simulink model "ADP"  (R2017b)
settings: Solver=FixedStepDiscrete  StartTime=0.0  StopTime=10.0  FixedStep=0.01  RelTol=1e-3  EnableMultiTasking=on
undefined symbols (not defined in the file): ADP050_RUNTIME_MS, ADP195_RUNTIME_MS, ADP_CONST100_NUMB, ADP_CONST2147483648_NUMB, ADP_CONST3_NUMB, ADP_CONST80_NUMB, ASWTYPE_FALSE, ASWTYPE_TRUE, CcADP_ABMDiagKL15DelayTi_ms, CcADP_ObcCmdto0Ti_ms, Enum_ADPStopChgReq, Enum_ISPDischgReq, Enum_LDPCC2St, Enum_MSMBMUState, Enum_ODPCCState, Enum_UDSPrjSel
libraries: AIWAYS_Powertrain_BMS_lib x68
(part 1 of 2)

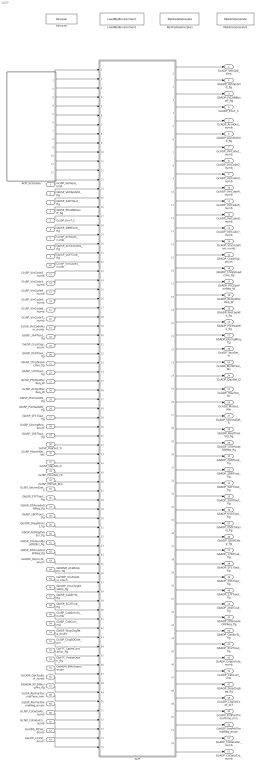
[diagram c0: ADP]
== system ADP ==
  GcISP_VehSpd_kmh : Inport
  GbISP_VehSpdVld_flg : Inport  Port=2
  GbISP_2ADTiout_flg : Inport  Port=3
  GbISP_PtCANBusoff_flg : Inport  Port=4
  GcISP_EnvT_C : Inport  Port=5
  GbISP_2BBTiout_flg : Inport  Port=6
  GcISP_AcmDist_numb : Inport  Port=7
  GbISP_AcmDistVld_flg : Inport  Port=8
  GbISP_2DFTiout_flg : Inport  Port=9
  GcISP_VinCode1_numb : Inport  Port=10
  GcISP_VinCode2_numb : Inport  Port=11
  GcISP_VinCode3_numb : Inport  Port=12
  GcISP_VinCode4_numb : Inport  Port=13
  GcISP_VinCode5_numb : Inport  Port=14
  GcISP_VinCode6_numb : Inport  Port=15
  GcISP_VinCode7_numb : Inport  Port=16
  GcISP_VinCodeNum_numb : Inport  Port=17
  GbISP_3AATiout_flg : Inport  Port=18
  GeISP_CrashSgl_enum : Inport  Port=19
  GbISP_050Tiout_flg : Inport  Port=20
  GbISP_ChrgStopActive_flg : Inport  Port=21
  GbISP_17DTiout_flg : Inport  Port=22
  GcISP_PTCOptPwrReq_W : Inport  Port=23
  GcISP_ACOptPwrReq_W : Inport  Port=24
  GbISP_PreCoolWk_flg : Inport  Port=25
  GbISP_PreHeatWk_flg : Inport  Port=26
  GbISP_2F1Tiout_flg : Inport  Port=27
  GeISP_DischgReq_enum : Inport  Port=28
  GbISP_195Tiout_flg : Inport  Port=29
  GcISP_YearSet_Yr : Inport  Port=30
  GcISP_MonthSet_Mn : Inport  Port=31
  GcISP_DaySet_D : Inport  Port=32
  GcISP_HourSet_Hr : Inport  Port=33
  GcISP_MinSet_Min : Inport  Port=34
  GcISP_SecondSet_S : Inport  Port=35
  GbISP_37FTiout_flg : Inport  Port=36
  GbISP_OTAmodeONReq_flg : Inport  Port=37
  GbISP_28DTiout_flg : Inport  Port=38
  GbVDP_DiagPermit_flg : Inport  Port=39
  GbISP_RcMsg050Err_flg : Inport  Port=40
  GbISP_ChkSumMsg050Err_flg : Inport  Port=41
  GbISP_OTAmodeOFFReq_flg : Inport  Port=42
  GeODP_ObcCcSt_enum : Inport  Port=43
  GbWSM_ACWkUpPrs_flg : Inport  Port=44
  GeVDP_VcuFalutLvl_enum : Inport  Port=45
  GbVDP_VcuChrgDisable_flg : Inport  Port=46
  GbISP_CabErrSt_flg : Inport  Port=47
  GbISP_3C2Tiout_flg : Inport  Port=48
  GcISP_CabErrInfo_numb : Inport  Port=49
  GcISP_CabCurr_mA : Inport  Port=50
  GeISP_StopChgReq_enum : Inport  Port=51
  GcISP_ChgSOCset_pct : Inport  Port=52
  GbFTC_OpenContactor_flg : Inport  Port=53
  GbFTC_PowerDown_flg : Inport  Port=54
  GeMSM_BMUState_enum : Inport  Port=55
  GcODP_ObcFaultLvl_numb : Inport  Port=56
  GbWSM_Kl15WkUpPrs_flg : Inport  Port=57
  GcISP_RmPreThemalTime_min : Inport  Port=58
  GeISP_RmPreThemalReq_enum : Inport  Port=59
  GcISP_CsDataVer_numb : Inport  Port=60
  GcISP_CsDataCrc_numb : Inport  Port=61
  GeUDS_PrjSel_enum : Inport  Port=62
  GeLDP_CC2St_enum : Inport  Port=63
  ADP : Subsystem
  ADP_Schedule : Stateflow chart  TreatAsAtomicUnit=on
  LoadMptEnvironment : AIWAYS_Powertrain_BMS_lib/Config/LoadMptEnvironment  ProjectName=Comm  SuppierID=NewPlatformUAES
  MptA2LGenerate1 : AIWAYS_Powertrain_BMS_lib/Config/MptA2LGenerate  SystemSampleTime=-1
  MptCodeGenerate1 : AIWAYS_Powertrain_BMS_lib/Config/MptCodeGenerate  SystemSampleTime=-1
  Revision : AIWAYS_Powertrain_BMS_lib/Config/Revision  curVersion='M110C112'  newVersion='M110C112'
  GcADP_VehSpd_kmh : Outport
  GbADP_VehSpdVld_flg : Outport  Port=2
  GbADP_PtCANBusoff_flg : Outport  Port=3
  GcADP_EnvT_C : Outport  Port=4
  GcADP_AcmDist_numb : Outport  Port=5
  GbADP_AcmDistVld_flg : Outport  Port=6
  GcADP_VinCode1_numb : Outport  Port=7
  GcADP_VinCode2_numb : Outport  Port=8
  GcADP_VinCode3_numb : Outport  Port=9
  GcADP_VinCode4_numb : Outport  Port=10
  GcADP_VinCode5_numb : Outport  Port=11
  GcADP_VinCode6_numb : Outport  Port=12
  GcADP_VinCode7_numb : Outport  Port=13
  GcADP_VinCodeNum_numb : Outport  Port=14
  GeADP_CrashSgl_enum : Outport  Port=15
  GbADP_ChrgStopActive_flg : Outport  Port=16
  GcADP_PTCOptPwrReq_W : Outport  Port=17
  GcADP_ACOptPwrReq_W : Outport  Port=18
  GbADP_PreCoolWk_flg : Outport  Port=19
  GbADP_PreHeatWk_flg : Outport  Port=20
  GbADP_DischgReq_flg : Outport  Port=21
  GcADP_YearSet_Yr : Outport  Port=22
  GcADP_MonthSet_Mn : Outport  Port=23
  GcADP_DaySet_D : Outport  Port=24
  GcADP_HourSet_Hr : Outport  Port=25
  GcADP_MinSet_Min : Outport  Port=26
  GcADP_SecondSet_S : Outport  Port=27
  GbADP_RealTimeVld_flg : Outport  Port=28
  GbADP_OTAmodeONReq_flg : Outport  Port=29
  GbADP_2ADTiout_flg : Outport  Port=30
  GbADP_2BBTiout_flg : Outport  Port=31
  GbADP_2DFTiout_flg : Outport  Port=32
  GbADP_3AATiout_flg : Outport  Port=33
  GbADP_050Tiout_flg : Outport  Port=34
  GbADP_050ChkSum_flg : Outport  Port=35
  GbADP_050RCMsg_flg : Outport  Port=36
  GbADP_17DTiout_flg : Outport  Port=37
  GbADP_2F1Tiout_flg : Outport  Port=38
  GbADP_195Tiout_flg : Outport  Port=39
  GbADP_37FTiout_flg : Outport  Port=40
  GbADP_28DTiout_flg : Outport  Port=41
  GbADP_OTAmodeOFFReq_flg : Outport  Port=42
  GbADP_CabErrSt_flg : Outport  Port=43
  GbADP_3C2Tiout_flg : Outport  Port=44
  GcADP_CabErrInfo_numb : Outport  Port=45
  GcADP_CabCurr_mA : Outport  Port=46
  GbADP_StopChgReq_flg : Outport  Port=47
  GcADP_ChgSOCset_pct : Outport  Port=48
  GcADP_RmPreThemalTime_min : Outport  Port=49
  GeADP_RmPreThemalReq_enum : Outport  Port=50
  GcADP_CsDataVer_numb : Outport  Port=51
  GcADP_CsDataCrc_numb : Outport  Port=52
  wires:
  ADP/1(GcADP_VehSpd_kmh) -> GcADP_VehSpd_kmh/1
  ADP/2(GbADP_VehSpdVld_flg) -> GbADP_VehSpdVld_flg/1
  ADP/3(GbADP_PtCANBusoff_flg) -> GbADP_PtCANBusoff_flg/1
  ADP/4(GcADP_EnvT_C) -> GcADP_EnvT_C/1
  ADP/5(GcADP_AcmDist_numb) -> GcADP_AcmDist_numb/1
  ADP/6(GbADP_AcmDistVld_flg) -> GbADP_AcmDistVld_flg/1
  ADP/7(GcADP_VinCode1_numb) -> GcADP_VinCode1_numb/1
  ADP/8(GcADP_VinCode2_numb) -> GcADP_VinCode2_numb/1
  ADP/9(GcADP_VinCode3_numb) -> GcADP_VinCode3_numb/1
  ADP/10(GcADP_VinCode4_numb) -> GcADP_VinCode4_numb/1
  ADP/11(GcADP_VinCode5_numb) -> GcADP_VinCode5_numb/1
  ADP/12(GcADP_VinCode6_numb) -> GcADP_VinCode6_numb/1
  ADP/13(GcADP_VinCode7_numb) -> GcADP_VinCode7_numb/1
  ADP/14(GcADP_VinCodeNum_numb) -> GcADP_VinCodeNum_numb/1
  ADP/15(GeADP_CrashSgl_enum) -> GeADP_CrashSgl_enum/1
  ADP/16(GbADP_ChrgStopActive_flg) -> GbADP_ChrgStopActive_flg/1
  ADP/17(GcADP_PTCOptPwrReq_W) -> GcADP_PTCOptPwrReq_W/1
  ADP/18(GcADP_ACOptPwrReq_W) -> GcADP_ACOptPwrReq_W/1
  ADP/19(GbADP_PreCoolWk_flg) -> GbADP_PreCoolWk_flg/1
  ADP/20(GbADP_PreHeatWk_flg) -> GbADP_PreHeatWk_flg/1
  ADP/21(GbADP_DischgReq_flg) -> GbADP_DischgReq_flg/1
  ADP/22(GcADP_YearSet_Yr) -> GcADP_YearSet_Yr/1
  ADP/23(GcADP_MonthSet_Mn) -> GcADP_MonthSet_Mn/1
  ADP/24(GcADP_DaySet_D) -> GcADP_DaySet_D/1
  ADP/25(GcADP_HourSet_Hr) -> GcADP_HourSet_Hr/1
  ADP/26(GcADP_MinSet_Min) -> GcADP_MinSet_Min/1
  ADP/27(GcADP_SecondSet_S) -> GcADP_SecondSet_S/1
  ADP/28(GbADP_RealTimeVld_flg) -> GbADP_RealTimeVld_flg/1
  ADP/29(GbADP_OTAmodeONReq_flg) -> GbADP_OTAmodeONReq_flg/1
  ADP/30(GbADP_2ADTiout_flg) -> GbADP_2ADTiout_flg/1
  ADP/31(GbADP_2BBTiout_flg) -> GbADP_2BBTiout_flg/1
  ADP/32(GbADP_2DFTiout_flg) -> GbADP_2DFTiout_flg/1
  ADP/33(GbADP_3AATiout_flg) -> GbADP_3AATiout_flg/1
  ADP/34(GbADP_050Tiout_flg) -> GbADP_050Tiout_flg/1
  ADP/35(GbADP_050ChkSum_flg) -> GbADP_050ChkSum_flg/1
  ADP/36(GbADP_050RCMsg_flg) -> GbADP_050RCMsg_flg/1
  ADP/37(GbADP_17DTiout_flg) -> GbADP_17DTiout_flg/1
  ADP/38(GbADP_2F1Tiout_flg) -> GbADP_2F1Tiout_flg/1
  ADP/39(GbADP_195Tiout_flg) -> GbADP_195Tiout_flg/1
  ADP/40(GbADP_37FTiout_flg) -> GbADP_37FTiout_flg/1
  ADP/41(GbADP_28DTiout_flg) -> GbADP_28DTiout_flg/1
  ADP/42(GbADP_OTAmodeOFFReq_flg) -> GbADP_OTAmodeOFFReq_flg/1
  ADP/43(GbADP_CabErrSt_flg) -> GbADP_CabErrSt_flg/1
  ADP/44(GbADP_3C2Tiout_flg) -> GbADP_3C2Tiout_flg/1
  ADP/45(GcADP_CabErrInfo_numb) -> GcADP_CabErrInfo_numb/1
  ADP/46(GcADP_CabCurr_mA) -> GcADP_CabCurr_mA/1
  ADP_Schedule/1(ADP_2AD_100ms()) -> ADP/1(ADP_2AD_100ms)
  ADP_Schedule/2(ADP_2BB_100ms()) -> ADP/2(ADP_2BB_100ms)
  ADP_Schedule/3(ADP_2DF_100ms()) -> ADP/3(ADP_2DF_100ms)
  ADP_Schedule/4(ADP_3AA_1000ms()) -> ADP/4(ADP_3AA_1000ms)
  ADP_Schedule/5(ADP_050_10ms()) -> ADP/5(ADP_050_10ms)
  ADP_Schedule/6(ADP_17D_20ms()) -> ADP/6(ADP_17D_20ms)
  ADP_Schedule/7(ADP_2F1_100ms()) -> ADP/7(ADP_2F1_100ms)
  ADP_Schedule/8(ADP_195_20ms()) -> ADP/8(ADP_195_20ms)
  ADP_Schedule/9(ADP_37F_500ms()) -> ADP/9(ADP_37F_500ms)
  ADP_Schedule/10(ADP_28D_20ms()) -> ADP/10(ADP_28D_20ms)
  ADP_Schedule/11(ADP_3C2_10ms()) -> ADP/11(ADP_3C2_10ms)
  GcISP_VehSpd_kmh/1 -> ADP/13(GcISP_VehSpd_kmh)
  GbISP_VehSpdVld_flg/1 -> ADP/14(GbISP_VehSpdVld_flg)
  GbISP_2ADTiout_flg/1 -> ADP/15(GbISP_2ADTiout_flg)
  GbISP_PtCANBusoff_flg/1 -> ADP/16(GbISP_PtCANBusoff_flg)
  GcISP_EnvT_C/1 -> ADP/17(GcISP_EnvT_C)
  GbISP_2BBTiout_flg/1 -> ADP/18(GbISP_2BBTiout_flg)
  GcISP_AcmDist_numb/1 -> ADP/19(GcISP_AcmDist_numb)
  GbISP_AcmDistVld_flg/1 -> ADP/20(GbISP_AcmDistVld_flg)
  GbISP_2DFTiout_flg/1 -> ADP/21(GbISP_2DFTiout_flg)
  GcISP_VinCode1_numb/1 -> ADP/22(GcISP_VinCode1_numb)
  GcISP_VinCode2_numb/1 -> ADP/23(GcISP_VinCode2_numb)
  GcISP_VinCode3_numb/1 -> ADP/24(GcISP_VinCode3_numb)
  GcISP_VinCode4_numb/1 -> ADP/25(GcISP_VinCode4_numb)
  GcISP_VinCode5_numb/1 -> ADP/26(GcISP_VinCode5_numb)
  GcISP_VinCode6_numb/1 -> ADP/27(GcISP_VinCode6_numb)
  GcISP_VinCode7_numb/1 -> ADP/28(GcISP_VinCode7_numb)
  GcISP_VinCodeNum_numb/1 -> ADP/29(GcISP_VinCodeNum_numb)
  GbISP_3AATiout_flg/1 -> ADP/30(GbISP_3AATiout_flg)
  GeISP_CrashSgl_enum/1 -> ADP/31(GeISP_CrashSgl_enum)
  GbISP_050Tiout_flg/1 -> ADP/32(GbISP_050Tiout_flg)
  GbISP_ChrgStopActive_flg/1 -> ADP/33(GbISP_ChrgStopActive_flg)
  GbISP_17DTiout_flg/1 -> ADP/34(GbISP_17DTiout_flg)
  GcISP_PTCOptPwrReq_W/1 -> ADP/35(GcISP_PTCOptPwrReq_W)
  GcISP_ACOptPwrReq_W/1 -> ADP/36(GcISP_ACOptPwrReq_W)
  GbISP_PreCoolWk_flg/1 -> ADP/37(GbISP_PreCoolWk_flg)
  GbISP_PreHeatWk_flg/1 -> ADP/38(GbISP_PreHeatWk_flg)
  GbISP_2F1Tiout_flg/1 -> ADP/39(GbISP_2F1Tiout_flg)
  GeISP_DischgReq_enum/1 -> ADP/40(GeISP_DischgReq_enum)
  GbISP_195Tiout_flg/1 -> ADP/41(GbISP_195Tiout_flg)
  GcISP_YearSet_Yr/1 -> ADP/42(GcISP_YearSet_Yr)
  GcISP_MonthSet_Mn/1 -> ADP/43(GcISP_MonthSet_Mn)
  GcISP_DaySet_D/1 -> ADP/44(GcISP_DaySet_D)
  GcISP_HourSet_Hr/1 -> ADP/45(GcISP_HourSet_Hr)
  GcISP_MinSet_Min/1 -> ADP/46(GcISP_MinSet_Min)
  GcISP_SecondSet_S/1 -> ADP/47(GcISP_SecondSet_S)
  GbISP_37FTiout_flg/1 -> ADP/48(GbISP_37FTiout_flg)
  GbISP_OTAmodeONReq_flg/1 -> ADP/49(GbISP_OTAmodeONReq_flg)
  GbISP_28DTiout_flg/1 -> ADP/50(GbISP_28DTiout_flg)
  GbVDP_DiagPermit_flg/1 -> ADP/51(GbVDP_DiagPermit_flg)
  GbISP_RcMsg050Err_flg/1 -> ADP/52(GbISP_RcMsg050Err_flg)
  GbISP_ChkSumMsg050Err_flg/1 -> ADP/53(GbISP_ChkSumMsg050Err_flg)
  GbISP_OTAmodeOFFReq_flg/1 -> ADP/54(GbISP_OTAmodeOFFReq_flg)
  GeODP_ObcCcSt_enum/1 -> ADP/55(GeODP_ObcCcSt_enum)
  GbWSM_ACWkUpPrs_flg/1 -> ADP/56(GbWSM_ACWkUpPrs_flg)
  GeVDP_VcuFalutLvl_enum/1 -> ADP/57(GeVDP_VcuFalutLvl_enum)
  GbVDP_VcuChrgDisable_flg/1 -> ADP/58(GbVDP_VcuChrgDisable_flg)
  GbISP_CabErrSt_flg/1 -> ADP/59(GbISP_CabErrSt_flg)
  GbISP_3C2Tiout_flg/1 -> ADP/60(GbISP_3C2Tiout_flg)
  GcISP_CabErrInfo_numb/1 -> ADP/61(GcISP_CabErrInfo_numb)
  GcISP_CabCurr_mA/1 -> ADP/62(GcISP_CabCurr_mA)
  GeISP_StopChgReq_enum/1 -> ADP/63(GeISP_StopChgReq_enum)
  GcISP_ChgSOCset_pct/1 -> ADP/64(GcISP_ChgSOCset_pct)
  ADP/47(GbADP_StopChgReq_flg) -> GbADP_StopChgReq_flg/1
  ADP/48(GcADP_ChgSOCset_pct) -> GcADP_ChgSOCset_pct/1
  GbFTC_OpenContactor_flg/1 -> ADP/65(GbFTC_OpenContactor_flg)
  GbFTC_PowerDown_flg/1 -> ADP/66(GbFTC_PowerDown_flg)
  GeMSM_BMUState_enum/1 -> ADP/67(GeMSM_BMUState_enum)
  GcODP_ObcFaultLvl_numb/1 -> ADP/68(GcODP_ObcFaultLvl_numb)
  GbWSM_Kl15WkUpPrs_flg/1 -> ADP/69(GbWSM_Kl15WkUpPrs_flg)
  ADP/49(GcADP_RmPreThemalTime_min) -> GcADP_RmPreThemalTime_min/1
  ADP/50(GeADP_RmPreThemalReq_enum) -> GeADP_RmPreThemalReq_enum/1
  GcISP_RmPreThemalTime_min/1 -> ADP/70(GcISP_RmPreThemalTime_min)
  GeISP_RmPreThemalReq_enum/1 -> ADP/71(GeISP_RmPreThemalReq_enum)
  GcISP_CsDataVer_numb/1 -> ADP/72(GcISP_CsDataVer_numb)
  GcISP_CsDataCrc_numb/1 -> ADP/73(GcISP_CsDataCrc_numb)
  ADP/51(GcADP_CsDataVer_numb) -> GcADP_CsDataVer_numb/1
  ADP/52(GcADP_CsDataCrc_numb) -> GcADP_CsDataCrc_numb/1
  ADP_Schedule/12(ADP_3A0_10ms()) -> ADP/12(ADP_3A0_10ms)
  GeUDS_PrjSel_enum/1 -> ADP/74(GeUDS_PrjSel_enum)
  GeLDP_CC2St_enum/1 -> ADP/75(GeLDP_CC2St_enum)

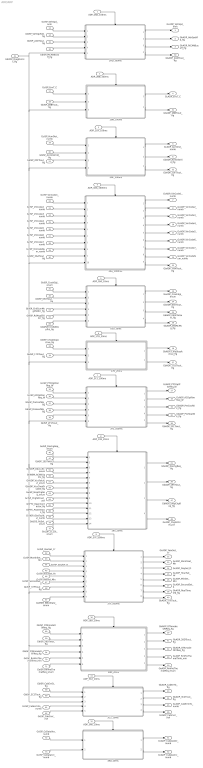
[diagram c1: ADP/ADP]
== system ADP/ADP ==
  ADP_2AD_100ms : Inport
  ADP_2BB_100ms : Inport  Port=2
  ADP_2DF_100ms : Inport  Port=3
  ADP_3AA_1000ms : Inport  Port=4
  ADP_050_10ms : Inport  Port=5
  ADP_17D_20ms : Inport  Port=6
  ADP_2F1_100ms : Inport  Port=7
  ADP_195_20ms : Inport  Port=8
  ADP_37F_500ms : Inport  Port=9
  ADP_28D_20ms : Inport  Port=10
  ADP_3C2_10ms : Inport  Port=11
  ADP_3A0_10ms : Inport  Port=12
  GcISP_VehSpd_kmh : Inport  Port=13
  GbISP_VehSpdVld_flg : Inport  Port=14
  GbISP_2ADTiout_flg : Inport  Port=15
  GbISP_PtCANBusoff_flg : Inport  Port=16
  GcISP_EnvT_C : Inport  Port=17
  GbISP_2BBTiout_flg : Inport  Port=18
  GcISP_AcmDist_numb : Inport  Port=19
  GbISP_AcmDistVld_flg : Inport  Port=20
  GbISP_2DFTiout_flg : Inport  Port=21
  GcISP_VinCode1_numb : Inport  Port=22
  GcISP_VinCode2_numb : Inport  Port=23
  GcISP_VinCode3_numb : Inport  Port=24
  GcISP_VinCode4_numb : Inport  Port=25
  GcISP_VinCode5_numb : Inport  Port=26
  GcISP_VinCode6_numb : Inport  Port=27
  GcISP_VinCode7_numb : Inport  Port=28
  GcISP_VinCodeNum_numb : Inport  Port=29
  GbISP_3AATiout_flg : Inport  Port=30
  GeISP_CrashSgl_enum : Inport  Port=31
  GbISP_050Tiout_flg : Inport  Port=32
  GbISP_ChrgStopActive_flg : Inport  Port=33
  GbISP_17DTiout_flg : Inport  Port=34
  GcISP_PTCOptPwrReq_W : Inport  Port=35
  GcISP_ACOptPwrReq_W : Inport  Port=36
  GbISP_PreCoolWk_flg : Inport  Port=37
  GbISP_PreHeatWk_flg : Inport  Port=38
  GbISP_2F1Tiout_flg : Inport  Port=39
  GeISP_DischgReq_enum : Inport  Port=40
  GbISP_195Tiout_flg : Inport  Port=41
  GcISP_YearSet_Yr : Inport  Port=42
  GcISP_MonthSet_Mn : Inport  Port=43
  GcISP_DaySet_D : Inport  Port=44
  GcISP_HourSet_Hr : Inport  Port=45
  GcISP_MinSet_Min : Inport  Port=46
  GcISP_SecondSet_S : Inport  Port=47
  GbISP_37FTiout_flg : Inport  Port=48
  GbISP_OTAmodeONReq_flg : Inport  Port=49
  GbISP_28DTiout_flg : Inport  Port=50
  GbVDP_DiagPermit_flg : Inport  Port=51
  GbISP_RcMsg050Err_flg : Inport  Port=52
  GbISP_ChkSumMsg050Err_flg : Inport  Port=53
  GbISP_OTAmodeOFFReq_flg : Inport  Port=54
  GeODP_ObcCcSt_enum : Inport  Port=55
  GbWSM_ACWkUpPrs_flg : Inport  Port=56
  GeVDP_VcuFalutLvl_enum : Inport  Port=57
  GbVDP_VcuChrgDisable_flg : Inport  Port=58
  GbISP_CabErrSt_flg : Inport  Port=59
  GbISP_3C2Tiout_flg : Inport  Port=60
  GcISP_CabErrInfo_numb : Inport  Port=61
  GcISP_CabCurr_mA : Inport  Port=62
  GeISP_StopChgReq_enum : Inport  Port=63
  GcISP_ChgSOCset_pct : Inport  Port=64
  GbFTC_OpenContactor_flg : Inport  Port=65
  GbFTC_PowerDown_flg : Inport  Port=66
  GeMSM_BMUState_enum : Inport  Port=67
  GcODP_ObcFaultLvl_numb : Inport  Port=68
  GbWSM_Kl15WkUpPrs_flg : Inport  Port=69
  GcISP_RmPreThemalTime_min : Inport  Port=70
  GeISP_RmPreThemalReq_enum : Inport  Port=71
  GcISP_CsDataVer_numb : Inport  Port=72
  GcISP_CsDataCrc_numb : Inport  Port=73
  GeUDS_PrjSel_enum : Inport  Port=74
  GeLDP_CC2St_enum : Inport  Port=75
  050_10ms : Subsystem
  17D_20ms : Subsystem
  195_20ms : Subsystem
  28D_20ms : Subsystem
  2AD_100ms : Subsystem
  2BB_100ms : Subsystem
  2DF_100ms : Subsystem
  2F1_100ms : Subsystem
  37F_500ms : Subsystem
  3A0_10ms : Subsystem
  3AA_1000ms : Subsystem
  3C2_10ms : Subsystem
  GcADP_VehSpd_kmh : Outport
  GbADP_VehSpdVld_flg : Outport  Port=2
  GbADP_PtCANBusoff_flg : Outport  Port=3
  GcADP_EnvT_C : Outport  Port=4
  GcADP_AcmDist_numb : Outport  Port=5
  GbADP_AcmDistVld_flg : Outport  Port=6
  GcADP_VinCode1_numb : Outport  Port=7
  GcADP_VinCode2_numb : Outport  Port=8
  GcADP_VinCode3_numb : Outport  Port=9
  GcADP_VinCode4_numb : Outport  Port=10
  GcADP_VinCode5_numb : Outport  Port=11
  GcADP_VinCode6_numb : Outport  Port=12
  GcADP_VinCode7_numb : Outport  Port=13
  GcADP_VinCodeNum_numb : Outport  Port=14
  GeADP_CrashSgl_enum : Outport  Port=15
  GbADP_ChrgStopActive_flg : Outport  Port=16
  GcADP_PTCOptPwrReq_W : Outport  Port=17
  GcADP_ACOptPwrReq_W : Outport  Port=18
  GbADP_PreCoolWk_flg : Outport  Port=19
  GbADP_PreHeatWk_flg : Outport  Port=20
  GbADP_DischgReq_flg : Outport  Port=21
  GcADP_YearSet_Yr : Outport  Port=22
  GcADP_MonthSet_Mn : Outport  Port=23
  GcADP_DaySet_D : Outport  Port=24
  GcADP_HourSet_Hr : Outport  Port=25
  GcADP_MinSet_Min : Outport  Port=26
  GcADP_SecondSet_S : Outport  Port=27
  GbADP_RealTimeVld_flg : Outport  Port=28
  GbADP_OTAmodeONReq_flg : Outport  Port=29
  GbADP_2ADTiout_flg : Outport  Port=30
  GbADP_2BBTiout_flg : Outport  Port=31
  GbADP_2DFTiout_flg : Outport  Port=32
  GbADP_3AATiout_flg : Outport  Port=33
  GbADP_050Tiout_flg : Outport  Port=34
  GbADP_050ChkSum_flg : Outport  Port=35
  GbADP_050RCMsg_flg : Outport  Port=36
  GbADP_17DTiout_flg : Outport  Port=37
  GbADP_2F1Tiout_flg : Outport  Port=38
  GbADP_195Tiout_flg : Outport  Port=39
  GbADP_37FTiout_flg : Outport  Port=40
  GbADP_28DTiout_flg : Outport  Port=41
  GbADP_OTAmodeOFFReq_flg : Outport  Port=42
  GbADP_CabErrSt_flg : Outport  Port=43
  GbADP_3C2Tiout_flg : Outport  Port=44
  GcADP_CabErrInfo_numb : Outport  Port=45
  GcADP_CabCurr_mA : Outport  Port=46
  GbADP_StopChgReq_flg : Outport  Port=47
  GcADP_ChgSOCset_pct : Outport  Port=48
  GcADP_RmPreThemalTime_min : Outport  Port=49
  GeADP_RmPreThemalReq_enum : Outport  Port=50
  GcADP_CsDataVer_numb : Outport  Port=51
  GcADP_CsDataCrc_numb : Outport  Port=52
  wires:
  ADP_2AD_100ms/1 -> 2AD_100ms/Trigger
  ADP_2BB_100ms/1 -> 2BB_100ms/Trigger
  ADP_2DF_100ms/1 -> 2DF_100ms/Trigger
  ADP_3AA_1000ms/1 -> 3AA_1000ms/Trigger
  ADP_050_10ms/1 -> 050_10ms/Trigger
  ADP_17D_20ms/1 -> 17D_20ms/Trigger
  ADP_2F1_100ms/1 -> 2F1_100ms/Trigger
  ADP_195_20ms/1 -> 195_20ms/Trigger
  ADP_37F_500ms/1 -> 37F_500ms/Trigger
  ADP_28D_20ms/1 -> 28D_20ms/Trigger
  GcISP_VehSpd_kmh/1 -> 2AD_100ms/1(GcISP_VehSpd_kmh)
  GbISP_VehSpdVld_flg/1 -> 2AD_100ms/2(GbISP_VehSpdVld_flg)
  GbISP_2ADTiout_flg/1 -> 2AD_100ms/3(GbISP_2ADTiout_flg)
  GbISP_PtCANBusoff_flg/1 -> 2AD_100ms/4(GbISP_PtCANBusoff_flg)
  2AD_100ms/1(GcADP_VehSpd_kmh) -> GcADP_VehSpd_kmh/1
  2AD_100ms/2(GbADP_VehSpdVld_flg) -> GbADP_VehSpdVld_flg/1
  2AD_100ms/3(GbADP_PtCANBusoff_flg) -> GbADP_PtCANBusoff_flg/1
  2BB_100ms/1(GcADP_EnvT_C) -> GcADP_EnvT_C/1
  GbISP_2BBTiout_flg/1 -> 2BB_100ms/2(GbISP_2BBTiout_flg)
  GcISP_EnvT_C/1 -> 2BB_100ms/1(GcISP_EnvT_C)
  GcISP_AcmDist_numb/1 -> 2DF_100ms/1(GcISP_AcmDist_numb)
  GbISP_AcmDistVld_flg/1 -> 2DF_100ms/2(GbISP_AcmDistVld_flg)
  GbISP_2DFTiout_flg/1 -> 2DF_100ms/3(GbISP_2DFTiout_flg)
  2DF_100ms/1(GcADP_AcmDist_numb) -> GcADP_AcmDist_numb/1
  2DF_100ms/2(GbADP_AcmDistVld_flg) -> GbADP_AcmDistVld_flg/1
  GcISP_VinCode1_numb/1 -> 3AA_1000ms/1(GcISP_VinCode1_numb)
  GcISP_VinCode2_numb/1 -> 3AA_1000ms/2(GcISP_VinCode2_numb)
  GcISP_VinCode3_numb/1 -> 3AA_1000ms/3(GcISP_VinCode3_numb)
  GcISP_VinCode4_numb/1 -> 3AA_1000ms/4(GcISP_VinCode4_numb)
  GcISP_VinCode5_numb/1 -> 3AA_1000ms/5(GcISP_VinCode5_numb)
  GcISP_VinCode6_numb/1 -> 3AA_1000ms/6(GcISP_VinCode6_numb)
  GcISP_VinCode7_numb/1 -> 3AA_1000ms/7(GcISP_VinCode7_numb)
  GcISP_VinCodeNum_numb/1 -> 3AA_1000ms/8(GcISP_VinCodeNum_numb)
  GbISP_3AATiout_flg/1 -> 3AA_1000ms/9(GbISP_3AATiout_flg)
  3AA_1000ms/1(GcADP_VinCode1_numb) -> GcADP_VinCode1_numb/1
  3AA_1000ms/2(GcADP_VinCode2_numb) -> GcADP_VinCode2_numb/1
  3AA_1000ms/3(GcADP_VinCode3_numb) -> GcADP_VinCode3_numb/1
  3AA_1000ms/4(GcADP_VinCode4_numb) -> GcADP_VinCode4_numb/1
  3AA_1000ms/5(GcADP_VinCode5_numb) -> GcADP_VinCode5_numb/1
  3AA_1000ms/6(GcADP_VinCode6_numb) -> GcADP_VinCode6_numb/1
  3AA_1000ms/7(GcADP_VinCode7_numb) -> GcADP_VinCode7_numb/1
  3AA_1000ms/8(GcADP_VinCodeNum_numb) -> GcADP_VinCodeNum_numb/1
  GeISP_CrashSgl_enum/1 -> 050_10ms/1(GeISP_CrashSgl_enum)
  GbISP_050Tiout_flg/1 -> 050_10ms/2(GbISP_050Tiout_flg)
  050_10ms/1(GeADP_CrashSgl_enum) -> GeADP_CrashSgl_enum/1
  GbISP_ChrgStopActive_flg/1 -> 17D_20ms/1(GbISP_ChrgStopActive_flg)
  17D_20ms/1(GbADP_ChrgStopActive_flg) -> GbADP_ChrgStopActive_flg/1
  GbISP_17DTiout_flg/1 -> 17D_20ms/2(GbISP_17DTiout_flg)
  GcISP_PTCOptPwrReq_W/1 -> 2F1_100ms/1(GcISP_PTCOptPwrReq_W)
  GcISP_ACOptPwrReq_W/1 -> 2F1_100ms/2(GcISP_ACOptPwrReq_W)
  GbISP_PreCoolWk_flg/1 -> 2F1_100ms/3(GbISP_PreCoolWk_flg)
  GbISP_PreHeatWk_flg/1 -> 2F1_100ms/4(GbISP_PreHeatWk_flg)
  GbISP_2F1Tiout_flg/1 -> 2F1_100ms/5(GbISP_2F1Tiout_flg)
  2F1_100ms/2(GcADP_ACOptPwrReq_W) -> GcADP_ACOptPwrReq_W/1
  2F1_100ms/1(GcADP_PTCOptPwrReq_W) -> GcADP_PTCOptPwrReq_W/1
  2F1_100ms/3(GbADP_PreCoolWk_flg) -> GbADP_PreCoolWk_flg/1
  2F1_100ms/4(GbADP_PreHeatWk_flg) -> GbADP_PreHeatWk_flg/1
  GeISP_DischgReq_enum/1 -> 195_20ms/1(GeISP_DischgReq_enum)
  GbISP_195Tiout_flg/1 -> 195_20ms/2(GbISP_195Tiout_flg)
  195_20ms/1(GbADP_DischgReq_flg) -> GbADP_DischgReq_flg/1
  GcISP_YearSet_Yr/1 -> 37F_500ms/1(GcISP_YearSet_Yr)
  GcISP_MonthSet_Mn/1 -> 37F_500ms/2(GcISP_MonthSet_Mn)
  GcISP_DaySet_D/1 -> 37F_500ms/3(GcISP_DaySet_D)
  GcISP_HourSet_Hr/1 -> 37F_500ms/4(GcISP_HourSet_Hr)
  GcISP_MinSet_Min/1 -> 37F_500ms/5(GcISP_MinSet_Min)
  GcISP_SecondSet_S/1 -> 37F_500ms/6(GcISP_SecondSet_S)
  GbISP_37FTiout_flg/1 -> 37F_500ms/7(GbISP_37FTiout_flg)
  37F_500ms/1(GcADP_YearSet_Yr) -> GcADP_YearSet_Yr/1
  37F_500ms/2(GcADP_MonthSet_Mn) -> GcADP_MonthSet_Mn/1
  37F_500ms/3(GcADP_DaySet_D) -> GcADP_DaySet_D/1
  37F_500ms/4(GcADP_HourSet_Hr) -> GcADP_HourSet_Hr/1
  37F_500ms/5(GcADP_MinSet_Min) -> GcADP_MinSet_Min/1
  37F_500ms/6(GcADP_SecondSet_S) -> GcADP_SecondSet_S/1
  37F_500ms/7(GbADP_RealTimeVld_flg) -> GbADP_RealTimeVld_flg/1
  GbISP_OTAmodeONReq_flg/1 -> 28D_20ms/1(GbISP_OTAmodeONReq_flg)
  GbISP_28DTiout_flg/1 -> 28D_20ms/2(GbISP_28DTiout_flg)
  28D_20ms/1(GbADP_OTAmodeONReq_flg) -> GbADP_OTAmodeONReq_flg/1
  2AD_100ms/4(GbADP_2ADTiout_flg) -> GbADP_2ADTiout_flg/1
  GbVDP_DiagPermit_flg/1 -> 2AD_100ms/5(GbVDP_DiagPermit_flg), 3C2_10ms/3(GbVDP_DiagPermit_flg), 28D_20ms/3(GbVDP_DiagPermit_flg), 37F_500ms/8(GbVDP_DiagPermit_flg), 195_20ms/3(GbVDP_DiagPermit_flg), 2F1_100ms/6(GbVDP_DiagPermit_flg), 17D_20ms/3(GbVDP_DiagPermit_flg), 050_10ms/3(GbVDP_DiagPermit_flg), 3AA_1000ms/10(GbVDP_DiagPermit_flg), 2DF_100ms/4(GbVDP_DiagPermit_flg), 2BB_100ms/3(GbVDP_DiagPermit_flg)
  2BB_100ms/2(GbADP_2BBTiout_flg) -> GbADP_2BBTiout_flg/1
  2DF_100ms/3(GbADP_2DFTiout_flg) -> GbADP_2DFTiout_flg/1
  3AA_1000ms/9(GbADP_3AATiout_flg) -> GbADP_3AATiout_flg/1
  GbISP_RcMsg050Err_flg/1 -> 050_10ms/5(GbISP_RcMsg050Err_flg)
  GbISP_ChkSumMsg050Err_flg/1 -> 050_10ms/4(GbISP_ChkSumMsg050Err_flg)
  050_10ms/2(GbADP_050Tiout_flg) -> GbADP_050Tiout_flg/1
  050_10ms/3(GbADP_050ChkSum_flg) -> GbADP_050ChkSum_flg/1
  050_10ms/4(GbADP_050RCMsg_flg) -> GbADP_050RCMsg_flg/1
  17D_20ms/2(GbADP_17DTiout_flg) -> GbADP_17DTiout_flg/1
  2F1_100ms/5(GbADP_2F1Tiout_flg) -> GbADP_2F1Tiout_flg/1
  195_20ms/2(GbADP_195Tiout_flg) -> GbADP_195Tiout_flg/1
  37F_500ms/8(GbADP_37FTiout_flg) -> GbADP_37FTiout_flg/1
  28D_20ms/2(GbADP_28DTiout_flg) -> GbADP_28DTiout_flg/1
  GbISP_OTAmodeOFFReq_flg/1 -> 28D_20ms/4(GbISP_OTAmodeOFFReq_flg)
  28D_20ms/3(GbADP_OTAmodeOFFReq_flg) -> GbADP_OTAmodeOFFReq_flg/1
  GbWSM_ACWkUpPrs_flg/1 -> 195_20ms/5(GbWSM_ACWkUpPrs_flg)
  GeODP_ObcCcSt_enum/1 -> 195_20ms/4(GeODP_ObcCcSt_enum)
  GbVDP_VcuChrgDisable_flg/1 -> 195_20ms/7(GbVDP_VcuChrgDisable_flg)
  GeVDP_VcuFalutLvl_enum/1 -> 195_20ms/6(GeVDP_VcuFalutLvl_enum)
  ADP_3C2_10ms/1 -> 3C2_10ms/Trigger
  GbISP_CabErrSt_flg/1 -> 3C2_10ms/1(GbISP_CabErrSt_flg)
  GbISP_3C2Tiout_flg/1 -> 3C2_10ms/2(GbISP_3C2Tiout_flg)
  GcISP_CabErrInfo_numb/1 -> 3C2_10ms/4(GcISP_CabErrInfo_numb)
  3C2_10ms/1(GbADP_CabErrSt_flg) -> GbADP_CabErrSt_flg/1
  3C2_10ms/2(GbADP_3C2Tiout_flg) -> GbADP_3C2Tiout_flg/1
  3C2_10ms/3(GcADP_CabErrInfo_numb) -> GcADP_CabErrInfo_numb/1
  GcISP_CabCurr_mA/1 -> 3C2_10ms/5(GcISP_CabCurr_mA)
  3C2_10ms/4(GcADP_CabCurr_mA) -> GcADP_CabCurr_mA/1
  GeISP_StopChgReq_enum/1 -> 195_20ms/8(GeISP_StopChgReq_enum)
  GcISP_ChgSOCset_pct/1 -> 195_20ms/9(GcISP_ChgSOCset_pct)
  195_20ms/3(GbADP_StopChgReq_flg) -> GbADP_StopChgReq_flg/1
  195_20ms/4(GcADP_ChgSOCset_pct) -> GcADP_ChgSOCset_pct/1
  GbFTC_OpenContactor_flg/1 -> 195_20ms/10(GbFTC_OpenContactor_flg)
  GbFTC_PowerDown_flg/1 -> 195_20ms/11(GbFTC_PowerDown_flg)
  GeMSM_BMUState_enum/1 -> 37F_500ms/9(GeMSM_BMUState_enum)
  GcODP_ObcFaultLvl_numb/1 -> 195_20ms/12(GcODP_ObcFaultLvl_numb)
  GbWSM_Kl15WkUpPrs_flg/1 -> 050_10ms/6(GbWSM_Kl15WkUpPrs_flg)
  GcISP_RmPreThemalTime_min/1 -> 28D_20ms/5(GcISP_RmPreThemalTime_min)
  GeISP_RmPreThemalReq_enum/1 -> 28D_20ms/6(GeISP_RmPreThemalReq_enum)
  28D_20ms/4(GcADP_RmPreThemalTime_min) -> GcADP_RmPreThemalTime_min/1
  28D_20ms/5(GeADP_RmPreThemalReq_enum) -> GeADP_RmPreThemalReq_enum/1
  ADP_3A0_10ms/1 -> 3A0_10ms/Trigger
  GcISP_CsDataVer_numb/1 -> 3A0_10ms/1(GcISP_CsDataVer_numb)
  GcISP_CsDataCrc_numb/1 -> 3A0_10ms/2(GcISP_CsDataCrc_numb)
  3A0_10ms/1(GcADP_CsDataVer_numb) -> GcADP_CsDataVer_numb/1
  3A0_10ms/2(GcADP_CsDataCrc_numb) -> GcADP_CsDataCrc_numb/1
  GeUDS_PrjSel_enum/1 -> 195_20ms/13(GeUDS_PrjSel_enum)
  GeLDP_CC2St_enum/1 -> 195_20ms/14(GeLDP_CC2St_enum)

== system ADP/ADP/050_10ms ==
  GeISP_CrashSgl_enum : Inport
  GbISP_050Tiout_flg : Inport  Port=2
  GbVDP_DiagPermit_flg : Inport  Port=3
  GbISP_ChkSumMsg050Err_flg : Inport  Port=4
  GbISP_RcMsg050Err_flg : Inport  Port=5
  GbWSM_Kl15WkUpPrs_flg : Inport  Port=6
  ADP_050_10ms : TriggerPort  TriggerType=function-call  VariantControl=(inherit)
  050_10ms_sys : Subsystem
  GeADP_CrashSgl_enum : Outport
  GbADP_050Tiout_flg : Outport  Port=2
  GbADP_050ChkSum_flg : Outport  Port=3
  GbADP_050RCMsg_flg : Outport  Port=4
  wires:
  GeISP_CrashSgl_enum/1 -> 050_10ms_sys/1(GeISP_CrashSgl_enum)
  GbISP_050Tiout_flg/1 -> 050_10ms_sys/2(GbISP_050Tiout_flg)
  050_10ms_sys/1(GeADP_CrashSgl_enum) -> GeADP_CrashSgl_enum/1
  050_10ms_sys/2(GbADP_050Tiout_flg) -> GbADP_050Tiout_flg/1
  050_10ms_sys/3(GbADP_050ChkSum_flg) -> GbADP_050ChkSum_flg/1
  050_10ms_sys/4(GbADP_050RCMsg_flg) -> GbADP_050RCMsg_flg/1
  GbVDP_DiagPermit_flg/1 -> 050_10ms_sys/3(GbVDP_DiagPermit_flg)
  GbISP_ChkSumMsg050Err_flg/1 -> 050_10ms_sys/4(GbISP_ChkSumMsg050Err_flg)
  GbISP_RcMsg050Err_flg/1 -> 050_10ms_sys/5(GbISP_RcMsg050Err_flg)
  GbWSM_Kl15WkUpPrs_flg/1 -> 050_10ms_sys/6(GbWSM_Kl15WkUpPrs_flg)

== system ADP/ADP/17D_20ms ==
  GbISP_ChrgStopActive_flg : Inport
  GbISP_17DTiout_flg : Inport  Port=2
  GbVDP_DiagPermit_flg : Inport  Port=3
  ADP_17D_20ms : TriggerPort  TriggerType=function-call  VariantControl=(inherit)
  17D_20ms_sys : Subsystem
  GbADP_ChrgStopActive_flg : Outport
  GbADP_17DTiout_flg : Outport  Port=2
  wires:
  GbISP_ChrgStopActive_flg/1 -> 17D_20ms_sys/1(GbISP_ChrgStopActive_flg)
  GbISP_17DTiout_flg/1 -> 17D_20ms_sys/2(GbISP_17DTiout_flg)
  17D_20ms_sys/1(GbADP_ChrgStopActive_flg) -> GbADP_ChrgStopActive_flg/1
  GbVDP_DiagPermit_flg/1 -> 17D_20ms_sys/3(GbVDP_DiagPermit_flg)
  17D_20ms_sys/2(GbADP_17DTiout_flg) -> GbADP_17DTiout_flg/1

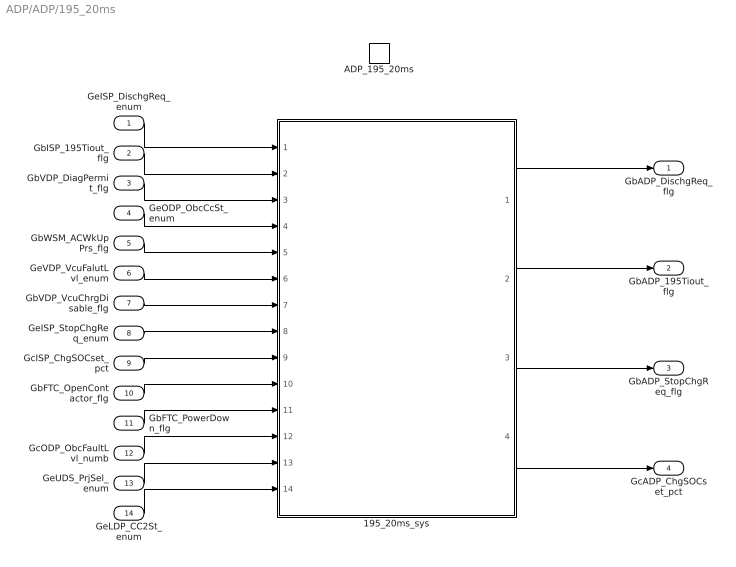
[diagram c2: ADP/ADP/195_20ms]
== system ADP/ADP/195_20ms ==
  GeISP_DischgReq_enum : Inport
  GbISP_195Tiout_flg : Inport  Port=2
  GbVDP_DiagPermit_flg : Inport  Port=3
  GeODP_ObcCcSt_enum : Inport  Port=4
  GbWSM_ACWkUpPrs_flg : Inport  Port=5
  GeVDP_VcuFalutLvl_enum : Inport  Port=6
  GbVDP_VcuChrgDisable_flg : Inport  Port=7
  GeISP_StopChgReq_enum : Inport  Port=8
  GcISP_ChgSOCset_pct : Inport  Port=9
  GbFTC_OpenContactor_flg : Inport  Port=10
  GbFTC_PowerDown_flg : Inport  Port=11
  GcODP_ObcFaultLvl_numb : Inport  Port=12
  GeUDS_PrjSel_enum : Inport  Port=13
  GeLDP_CC2St_enum : Inport  Port=14
  ADP_195_20ms : TriggerPort  TriggerType=function-call  VariantControl=(inherit)
  195_20ms_sys : Subsystem
  GbADP_DischgReq_flg : Outport
  GbADP_195Tiout_flg : Outport  Port=2
  GbADP_StopChgReq_flg : Outport  Port=3
  GcADP_ChgSOCset_pct : Outport  Port=4
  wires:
  GeISP_DischgReq_enum/1 -> 195_20ms_sys/1(GeISP_DischgReq_enum)
  GbISP_195Tiout_flg/1 -> 195_20ms_sys/2(GbISP_195Tiout_flg)
  195_20ms_sys/1(GbADP_DischgReq_flg) -> GbADP_DischgReq_flg/1
  GbVDP_DiagPermit_flg/1 -> 195_20ms_sys/3(GbVDP_DiagPermit_flg)
  195_20ms_sys/2(GbADP_195Tiout_flg) -> GbADP_195Tiout_flg/1
  GeODP_ObcCcSt_enum/1 -> 195_20ms_sys/4(GeODP_ObcCcSt_enum)
  GbWSM_ACWkUpPrs_flg/1 -> 195_20ms_sys/5(GbWSM_ACWkUpPrs_flg)
  GeVDP_VcuFalutLvl_enum/1 -> 195_20ms_sys/6(GeVDP_VcuFalutLvl_enum)
  GbVDP_VcuChrgDisable_flg/1 -> 195_20ms_sys/7(GbVDP_VcuChrgDisable_flg)
  195_20ms_sys/3(GbADP_StopChgReq_flg) -> GbADP_StopChgReq_flg/1
  195_20ms_sys/4(GcADP_ChgSOCset_pct) -> GcADP_ChgSOCset_pct/1
  GeISP_StopChgReq_enum/1 -> 195_20ms_sys/8(GeISP_StopChgReq_enum)
  GcISP_ChgSOCset_pct/1 -> 195_20ms_sys/9(GcISP_ChgSOCset_pct)
  GbFTC_OpenContactor_flg/1 -> 195_20ms_sys/10(GbFTC_OpenContactor_flg)
  GbFTC_PowerDown_flg/1 -> 195_20ms_sys/11(GbFTC_PowerDown_flg)
  GcODP_ObcFaultLvl_numb/1 -> 195_20ms_sys/12(GcODP_ObcFaultLvl_numb)
  GeUDS_PrjSel_enum/1 -> 195_20ms_sys/13(GeUDS_PrjSel_enum)
  GeLDP_CC2St_enum/1 -> 195_20ms_sys/14(GeLDP_CC2St_enum)

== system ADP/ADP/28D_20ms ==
  GbISP_OTAmodeONReq_flg : Inport
  GbISP_28DTiout_flg : Inport  Port=2
  GbVDP_DiagPermit_flg : Inport  Port=3
  GbISP_OTAmodeOFFReq_flg : Inport  Port=4
  GcISP_RmPreThemalTime_min : Inport  Port=5
  GeISP_RmPreThemalReq_enum : Inport  Port=6
  ADP_28D_20ms : TriggerPort  TriggerType=function-call  VariantControl=(inherit)
  28D_20ms_sys : Subsystem
  GbADP_OTAmodeONReq_flg : Outport
  GbADP_28DTiout_flg : Outport  Port=2
  GbADP_OTAmodeOFFReq_flg : Outport  Port=3
  GcADP_RmPreThemalTime_min : Outport  Port=4
  GeADP_RmPreThemalReq_enum : Outport  Port=5
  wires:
  GbISP_OTAmodeONReq_flg/1 -> 28D_20ms_sys/1(GbISP_OTAmodeONReq_flg)
  GbISP_28DTiout_flg/1 -> 28D_20ms_sys/2(GbISP_28DTiout_flg)
  28D_20ms_sys/1(GbADP_OTAmodeONReq_flg) -> GbADP_OTAmodeONReq_flg/1
  GbVDP_DiagPermit_flg/1 -> 28D_20ms_sys/3(GbVDP_DiagPermit_flg)
  28D_20ms_sys/2(GbADP_28DTiout_flg) -> GbADP_28DTiout_flg/1
  28D_20ms_sys/3(GbADP_OTAmodeOFFReq_flg) -> GbADP_OTAmodeOFFReq_flg/1
  GbISP_OTAmodeOFFReq_flg/1 -> 28D_20ms_sys/4(GbISP_OTAmodeOFFReq_flg)
  GcISP_RmPreThemalTime_min/1 -> 28D_20ms_sys/5(GcISP_RmPreThemalTime_min)
  GeISP_RmPreThemalReq_enum/1 -> 28D_20ms_sys/6(GeISP_RmPreThemalReq_enum)
  28D_20ms_sys/4(GcADP_RmPreThemalTime_min) -> GcADP_RmPreThemalTime_min/1
  28D_20ms_sys/5(GeADP_RmPreThemalReq_enum) -> GeADP_RmPreThemalReq_enum/1

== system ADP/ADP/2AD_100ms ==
  GcISP_VehSpd_kmh : Inport
  GbISP_VehSpdVld_flg : Inport  Port=2
  GbISP_2ADTiout_flg : Inport  Port=3
  GbISP_PtCANBusoff_flg : Inport  Port=4
  GbVDP_DiagPermit_flg : Inport  Port=5
  ADP_2AD_100ms : TriggerPort  TriggerType=function-call  VariantControl=(inherit)
  2AD_100ms_sys : Subsystem
  GcADP_VehSpd_kmh : Outport
  GbADP_VehSpdVld_flg : Outport  Port=2
  GbADP_PtCANBusoff_flg : Outport  Port=3
  GbADP_2ADTiout_flg : Outport  Port=4
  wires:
  GcISP_VehSpd_kmh/1 -> 2AD_100ms_sys/1(GcISP_VehSpd_kmh)
  GbISP_VehSpdVld_flg/1 -> 2AD_100ms_sys/2(GbISP_VehSpdVld_flg)
  GbISP_2ADTiout_flg/1 -> 2AD_100ms_sys/3(GbISP_2ADTiout_flg)
  2AD_100ms_sys/1(GcADP_VehSpd_kmh) -> GcADP_VehSpd_kmh/1
  2AD_100ms_sys/2(GbADP_VehSpdVld_flg) -> GbADP_VehSpdVld_flg/1
  GbISP_PtCANBusoff_flg/1 -> 2AD_100ms_sys/4(GbISP_PtCANBusoff_flg)
  2AD_100ms_sys/3(GbADP_PtCANBusoff_flg) -> GbADP_PtCANBusoff_flg/1
  GbVDP_DiagPermit_flg/1 -> 2AD_100ms_sys/5(GbVDP_DiagPermit_flg)
  2AD_100ms_sys/4(GbADP_2ADTiout_flg) -> GbADP_2ADTiout_flg/1

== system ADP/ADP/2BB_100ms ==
  GcISP_EnvT_C : Inport
  GbISP_2BBTiout_flg : Inport  Port=2
  GbVDP_DiagPermit_flg : Inport  Port=3
  ADP_2BB_100ms : TriggerPort  TriggerType=function-call  VariantControl=(inherit)
  2BB_100ms_sys : Subsystem
  GcADP_EnvT_C : Outport
  GbADP_2BBTiout_flg : Outport  Port=2
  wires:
  GcISP_EnvT_C/1 -> 2BB_100ms_sys/1(GcISP_EnvT_C)
  GbISP_2BBTiout_flg/1 -> 2BB_100ms_sys/2(GbISP_2BBTiout_flg)
  2BB_100ms_sys/1(GcADP_EnvT_C) -> GcADP_EnvT_C/1
  GbVDP_DiagPermit_flg/1 -> 2BB_100ms_sys/3(GbVDP_DiagPermit_flg)
  2BB_100ms_sys/2(GbADP_2BBTiout_flg) -> GbADP_2BBTiout_flg/1

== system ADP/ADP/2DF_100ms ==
  GcISP_AcmDist_numb : Inport
  GbISP_AcmDistVld_flg : Inport  Port=2
  GbISP_2DFTiout_flg : Inport  Port=3
  GbVDP_DiagPermit_flg : Inport  Port=4
  ADP_2DF_100ms : TriggerPort  TriggerType=function-call  VariantControl=(inherit)
  2DF_100ms_sys : Subsystem
  GcADP_AcmDist_numb : Outport
  GbADP_AcmDistVld_flg : Outport  Port=2
  GbADP_2DFTiout_flg : Outport  Port=3
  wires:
  GbISP_2DFTiout_flg/1 -> 2DF_100ms_sys/3(GbISP_2DFTiout_flg)
  GbISP_AcmDistVld_flg/1 -> 2DF_100ms_sys/2(GbISP_AcmDistVld_flg)
  GcISP_AcmDist_numb/1 -> 2DF_100ms_sys/1(GcISP_AcmDist_numb)
  2DF_100ms_sys/2(GbADP_AcmDistVld_flg) -> GbADP_AcmDistVld_flg/1
  2DF_100ms_sys/1(GcADP_AcmDist_numb) -> GcADP_AcmDist_numb/1
  GbVDP_DiagPermit_flg/1 -> 2DF_100ms_sys/4(GbVDP_DiagPermit_flg)
  2DF_100ms_sys/3(GbADP_2DFTiout_flg) -> GbADP_2DFTiout_flg/1

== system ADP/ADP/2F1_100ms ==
  GcISP_PTCOptPwrReq_W : Inport
  GcISP_ACOptPwrReq_W : Inport  Port=2
  GbISP_PreCoolWk_flg : Inport  Port=3
  GbISP_PreHeatWk_flg : Inport  Port=4
  GbISP_2F1Tiout_flg : Inport  Port=5
  GbVDP_DiagPermit_flg : Inport  Port=6
  ADP_2F1_100ms : TriggerPort  TriggerType=function-call  VariantControl=(inherit)
  2F1_100ms_sys : Subsystem
  GcADP_PTCOptPwrReq_W : Outport
  GcADP_ACOptPwrReq_W : Outport  Port=2
  GbADP_PreCoolWk_flg : Outport  Port=3
  GbADP_PreHeatWk_flg : Outport  Port=4
  GbADP_2F1Tiout_flg : Outport  Port=5
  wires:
  GcISP_PTCOptPwrReq_W/1 -> 2F1_100ms_sys/1(GcISP_PTCOptPwrReq_W)
  GcISP_ACOptPwrReq_W/1 -> 2F1_100ms_sys/2(GcISP_ACOptPwrReq_W)
  GbISP_PreCoolWk_flg/1 -> 2F1_100ms_sys/3(GbISP_PreCoolWk_flg)
  GbISP_PreHeatWk_flg/1 -> 2F1_100ms_sys/4(GbISP_PreHeatWk_flg)
  GbISP_2F1Tiout_flg/1 -> 2F1_100ms_sys/5(GbISP_2F1Tiout_flg)
  2F1_100ms_sys/1(GcADP_PTCOptPwrReq_W) -> GcADP_PTCOptPwrReq_W/1
  2F1_100ms_sys/2(GcADP_ACOptPwrReq_W) -> GcADP_ACOptPwrReq_W/1
  2F1_100ms_sys/4(GbADP_PreHeatWk_flg) -> GbADP_PreHeatWk_flg/1
  2F1_100ms_sys/3(GbADP_PreCoolWk_flg) -> GbADP_PreCoolWk_flg/1
  GbVDP_DiagPermit_flg/1 -> 2F1_100ms_sys/6(GbVDP_DiagPermit_flg)
  2F1_100ms_sys/5(GbADP_2F1Tiout_flg) -> GbADP_2F1Tiout_flg/1

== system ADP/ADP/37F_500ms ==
  GcISP_YearSet_Yr : Inport
  GcISP_MonthSet_Mn : Inport  Port=2
  GcISP_DaySet_D : Inport  Port=3
  GcISP_HourSet_Hr : Inport  Port=4
  GcISP_MinSet_Min : Inport  Port=5
  GcISP_SecondSet_S : Inport  Port=6
  GbISP_37FTiout_flg : Inport  Port=7
  GbVDP_DiagPermit_flg : Inport  Port=8
  GeMSM_BMUState_enum : Inport  Port=9
  ADP_37F_500ms : TriggerPort  TriggerType=function-call  VariantControl=(inherit)
  37F_500ms_sys : Subsystem
  GcADP_YearSet_Yr : Outport
  GcADP_MonthSet_Mn : Outport  Port=2
  GcADP_DaySet_D : Outport  Port=3
  GcADP_HourSet_Hr : Outport  Port=4
  GcADP_MinSet_Min : Outport  Port=5
  GcADP_SecondSet_S : Outport  Port=6
  GbADP_RealTimeVld_flg : Outport  Port=7
  GbADP_37FTiout_flg : Outport  Port=8
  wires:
  GcISP_YearSet_Yr/1 -> 37F_500ms_sys/1(GcISP_YearSet_Yr)
  GcISP_MonthSet_Mn/1 -> 37F_500ms_sys/2(GcISP_MonthSet_Mn)
  GcISP_DaySet_D/1 -> 37F_500ms_sys/3(GcISP_DaySet_D)
  GcISP_HourSet_Hr/1 -> 37F_500ms_sys/4(GcISP_HourSet_Hr)
  GcISP_MinSet_Min/1 -> 37F_500ms_sys/5(GcISP_MinSet_Min)
  GcISP_SecondSet_S/1 -> 37F_500ms_sys/6(GcISP_SecondSet_S)
  GbISP_37FTiout_flg/1 -> 37F_500ms_sys/7(GbISP_37FTiout_flg)
  37F_500ms_sys/1(GcADP_YearSet_Yr) -> GcADP_YearSet_Yr/1
  37F_500ms_sys/2(GcADP_MonthSet_Mn) -> GcADP_MonthSet_Mn/1
  37F_500ms_sys/3(GcADP_DaySet_D) -> GcADP_DaySet_D/1
  37F_500ms_sys/4(GcADP_HourSet_Hr) -> GcADP_HourSet_Hr/1
  37F_500ms_sys/5(GcADP_MinSet_Min) -> GcADP_MinSet_Min/1
  37F_500ms_sys/6(GcADP_SecondSet_S) -> GcADP_SecondSet_S/1
  37F_500ms_sys/7(GbADP_RealTimeVld_flg) -> GbADP_RealTimeVld_flg/1
  GbVDP_DiagPermit_flg/1 -> 37F_500ms_sys/8(GbVDP_DiagPermit_flg)
  37F_500ms_sys/8(GbADP_37FTiout_flg) -> GbADP_37FTiout_flg/1
  GeMSM_BMUState_enum/1 -> 37F_500ms_sys/9(GeMSM_BMUState_enum)

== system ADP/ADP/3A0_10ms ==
  GcISP_CsDataVer_numb : Inport
  GcISP_CsDataCrc_numb : Inport  Port=2
  ADP_3A0_10ms : TriggerPort  TriggerType=function-call  VariantControl=(inherit)
  3A0_10ms_sys : Subsystem
  GcADP_CsDataVer_numb : Outport
  GcADP_CsDataCrc_numb : Outport  Port=2
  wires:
  GcISP_CsDataVer_numb/1 -> 3A0_10ms_sys/1(GcISP_CsDataVer_numb)
  3A0_10ms_sys/1(GcADP_CsDataVer_numb) -> GcADP_CsDataVer_numb/1
  3A0_10ms_sys/2(GcADP_CsDataCrc_numb) -> GcADP_CsDataCrc_numb/1
  GcISP_CsDataCrc_numb/1 -> 3A0_10ms_sys/2(GcISP_CsDataCrc_numb)

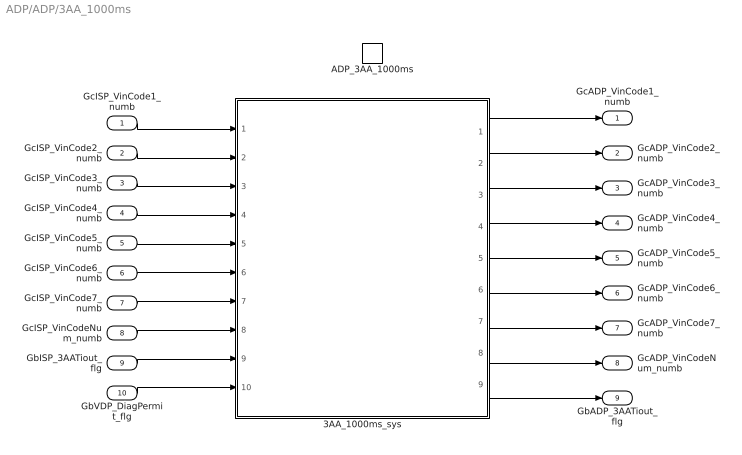
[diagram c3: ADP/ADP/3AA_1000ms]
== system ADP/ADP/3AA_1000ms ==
  GcISP_VinCode1_numb : Inport
  GcISP_VinCode2_numb : Inport  Port=2
  GcISP_VinCode3_numb : Inport  Port=3
  GcISP_VinCode4_numb : Inport  Port=4
  GcISP_VinCode5_numb : Inport  Port=5
  GcISP_VinCode6_numb : Inport  Port=6
  GcISP_VinCode7_numb : Inport  Port=7
  GcISP_VinCodeNum_numb : Inport  Port=8
  GbISP_3AATiout_flg : Inport  Port=9
  GbVDP_DiagPermit_flg : Inport  Port=10
  ADP_3AA_1000ms : TriggerPort  TriggerType=function-call  VariantControl=(inherit)
  3AA_1000ms_sys : Subsystem
  GcADP_VinCode1_numb : Outport
  GcADP_VinCode2_numb : Outport  Port=2
  GcADP_VinCode3_numb : Outport  Port=3
  GcADP_VinCode4_numb : Outport  Port=4
  GcADP_VinCode5_numb : Outport  Port=5
  GcADP_VinCode6_numb : Outport  Port=6
  GcADP_VinCode7_numb : Outport  Port=7
  GcADP_VinCodeNum_numb : Outport  Port=8
  GbADP_3AATiout_flg : Outport  Port=9
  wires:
  GcISP_VinCode1_numb/1 -> 3AA_1000ms_sys/1(GcISP_VinCode1_numb)
  GcISP_VinCode2_numb/1 -> 3AA_1000ms_sys/2(GcISP_VinCode2_numb)
  GcISP_VinCode3_numb/1 -> 3AA_1000ms_sys/3(GcISP_VinCode3_numb)
  GcISP_VinCode4_numb/1 -> 3AA_1000ms_sys/4(GcISP_VinCode4_numb)
  GcISP_VinCode5_numb/1 -> 3AA_1000ms_sys/5(GcISP_VinCode5_numb)
  GcISP_VinCode6_numb/1 -> 3AA_1000ms_sys/6(GcISP_VinCode6_numb)
  GcISP_VinCode7_numb/1 -> 3AA_1000ms_sys/7(GcISP_VinCode7_numb)
  GcISP_VinCodeNum_numb/1 -> 3AA_1000ms_sys/8(GcISP_VinCodeNum_numb)
  GbISP_3AATiout_flg/1 -> 3AA_1000ms_sys/9(GbISP_3AATiout_flg)
  3AA_1000ms_sys/1(GcADP_VinCode1_numb) -> GcADP_VinCode1_numb/1
  3AA_1000ms_sys/2(GcADP_VinCode2_numb) -> GcADP_VinCode2_numb/1
  3AA_1000ms_sys/3(GcADP_VinCode3_numb) -> GcADP_VinCode3_numb/1
  3AA_1000ms_sys/4(GcADP_VinCode4_numb) -> GcADP_VinCode4_numb/1
  3AA_1000ms_sys/5(GcADP_VinCode5_numb) -> GcADP_VinCode5_numb/1
  3AA_1000ms_sys/6(GcADP_VinCode6_numb) -> GcADP_VinCode6_numb/1
  3AA_1000ms_sys/7(GcADP_VinCode7_numb) -> GcADP_VinCode7_numb/1
  3AA_1000ms_sys/8(GcADP_VinCodeNum_numb) -> GcADP_VinCodeNum_numb/1
  GbVDP_DiagPermit_flg/1 -> 3AA_1000ms_sys/10(GbVDP_DiagPermit_flg)
  3AA_1000ms_sys/9(GbADP_3AATiout_flg) -> GbADP_3AATiout_flg/1

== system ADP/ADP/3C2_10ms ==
  GbISP_CabErrSt_flg : Inport
  GbISP_3C2Tiout_flg : Inport  Port=2
  GbVDP_DiagPermit_flg : Inport  Port=3
  GcISP_CabErrInfo_numb : Inport  Port=4
  GcISP_CabCurr_mA : Inport  Port=5
  ADP_3C2_10ms : TriggerPort  TriggerType=function-call  VariantControl=(inherit)
  3C2_10ms_sys : Subsystem
  GbADP_CabErrSt_flg : Outport
  GbADP_3C2Tiout_flg : Outport  Port=2
  GcADP_CabErrInfo_numb : Outport  Port=3
  GcADP_CabCurr_mA : Outport  Port=4
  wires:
  GcISP_CabErrInfo_numb/1 -> 3C2_10ms_sys/4(GcISP_CabErrInfo_numb)
  3C2_10ms_sys/3(GcADP_CabErrInfo_numb) -> GcADP_CabErrInfo_numb/1
  3C2_10ms_sys/2(GbADP_3C2Tiout_flg) -> GbADP_3C2Tiout_flg/1
  GbVDP_DiagPermit_flg/1 -> 3C2_10ms_sys/3(GbVDP_DiagPermit_flg)
  3C2_10ms_sys/1(GbADP_CabErrSt_flg) -> GbADP_CabErrSt_flg/1
  GbISP_3C2Tiout_flg/1 -> 3C2_10ms_sys/2(GbISP_3C2Tiout_flg)
  GbISP_CabErrSt_flg/1 -> 3C2_10ms_sys/1(GbISP_CabErrSt_flg)
  GcISP_CabCurr_mA/1 -> 3C2_10ms_sys/5(GcISP_CabCurr_mA)
  3C2_10ms_sys/4(GcADP_CabCurr_mA) -> GcADP_CabCurr_mA/1

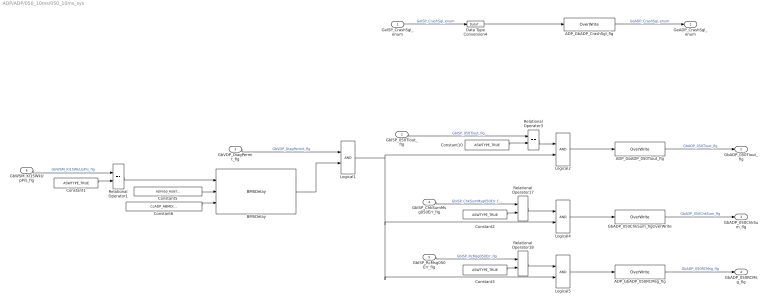
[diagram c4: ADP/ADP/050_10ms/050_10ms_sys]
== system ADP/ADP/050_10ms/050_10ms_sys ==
  GeISP_CrashSgl_enum : Inport
  GbISP_050Tiout_flg : Inport  Port=2
  GbVDP_DiagPermit_flg : Inport  Port=3
  GbISP_ChkSumMsg050Err_flg : Inport  Port=4
  GbISP_RcMsg050Err_flg : Inport  Port=5
  GbWSM_Kl15WkUpPrs_flg : Inport  Port=6
  ADP_GbADP_050RCMsg_flg : AIWAYS_Powertrain_BMS_lib/Signals/OverWrite  OverWrite_Value=CbADP_050RCMsgOvr_flg  OverWrite_flag=CbADP_050RCMsgOvrSwt_flg
  ADP_GbADP_050Tiout_flg : AIWAYS_Powertrain_BMS_lib/Signals/OverWrite  OverWrite_Value=CbADP_050TioutOvr_flg  OverWrite_flag=CbADP_050TioutOvrSwt_flg
  ADP_GbADP_CrashSgl_flg : AIWAYS_Powertrain_BMS_lib/Signals/OverWrite  OverWrite_Value=CeADP_CrashSglOvr_enum  OverWrite_flag=CbADP_CrashSglOvrSwt_flg
  BMSDelay : AIWAYS_Powertrain_BMS_lib/Debounce & Delay/BMSDelay
  Constant{1..3,10} (4 alike) : Constant  Value=ASWTYPE_TRUE
  Constant5 : Constant  Value=ADP050_RUNTIME_MS
  Constant6 : Constant  Value=CcADP_ABMDiagKL15DelayTi_ms
  Data Type Conversion4 : DataTypeConversion
  GbADP_050ChkSum_flgOverWrite : AIWAYS_Powertrain_BMS_lib/Signals/OverWrite  OverWrite_Value=CbADP_050ChkSumOvr_flg  OverWrite_flag=CbADP_050ChkSumOvrSwt_flg
  Logical{1..2,4..5} (4 alike) : Logic  OutDataTypeStr=boolean
  Relational Operator{1,3,17..18} (4 alike) : RelationalOperator  Operator===  OutDataTypeStr=boolean
  GeADP_CrashSgl_enum : Outport
  GbADP_050Tiout_flg : Outport  Port=2
  GbADP_050ChkSum_flg : Outport  Port=3
  GbADP_050RCMsg_flg : Outport  Port=4
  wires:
  Data Type Conversion4/1 -> ADP_GbADP_CrashSgl_flg/1
  ADP_GbADP_CrashSgl_flg/1 -> GeADP_CrashSgl_enum/1  "GeADP_CrashSgl_enum"
  GbISP_050Tiout_flg/1 -> Relational Operator3/1  "GbISP_050Tiout_flg"
  GeISP_CrashSgl_enum/1 -> Data Type Conversion4/1  "GeISP_CrashSgl_enum"
  GbVDP_DiagPermit_flg/1 -> Logical1/1  "GbVDP_DiagPermit_flg"
  Logical2/1 -> ADP_GbADP_050Tiout_flg/1
  Constant10/1 -> Relational Operator3/2
  Relational Operator3/1 -> Logical2/1
  GbISP_RcMsg050Err_flg/1 -> Relational Operator18/1  "GbISP_RcMsg050Err_flg"
  Constant2/1 -> Relational Operator17/2
  GbISP_ChkSumMsg050Err_flg/1 -> Relational Operator17/1  "GbISP_ChkSumMsg050Err_flg"
  Relational Operator18/1 -> Logical5/1
  Constant3/1 -> Relational Operator18/2
  Logical4/1 -> GbADP_050ChkSum_flgOverWrite/1
  Logical5/1 -> ADP_GbADP_050RCMsg_flg/1
  Relational Operator17/1 -> Logical4/1
  ADP_GbADP_050Tiout_flg/1 -> GbADP_050Tiout_flg/1  "GbADP_050Tiout_flg"
  GbADP_050ChkSum_flgOverWrite/1 -> GbADP_050ChkSum_flg/1  "GbADP_050ChkSum_flg"
  ADP_GbADP_050RCMsg_flg/1 -> GbADP_050RCMsg_flg/1  "GbADP_050RCMsg_flg"
  Logical1/1 -> Logical5/2, Logical4/2, Logical2/2
  Constant1/1 -> Relational Operator1/2
  GbWSM_Kl15WkUpPrs_flg/1 -> Relational Operator1/1  "GbWSM_Kl15WkUpPrs_flg"
  Constant6/1 -> BMSDelay/3
  Relational Operator1/1 -> BMSDelay/1
  Constant5/1 -> BMSDelay/2
  BMSDelay/1 -> Logical1/2

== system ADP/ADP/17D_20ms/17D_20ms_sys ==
  GbISP_ChrgStopActive_flg : Inport
  GbISP_17DTiout_flg : Inport  Port=2
  GbVDP_DiagPermit_flg : Inport  Port=3
  ADP_GbADP_17DTiout_flg : AIWAYS_Powertrain_BMS_lib/Signals/OverWrite  OverWrite_Value=CbADP_17DTioutOvr_flg  OverWrite_flag=CbADP_17DTioutOvrSwt_flg
  ADP_GbADP_ChrgStopActive_flg : AIWAYS_Powertrain_BMS_lib/Signals/OverWrite  OverWrite_Value=CbADP_ChrgStopActiveOvr_flg  OverWrite_flag=CbADP_ChrgStopActiveOvrSwt_flg
  Constant1 : Constant  Value=ASWTYPE_FALSE
  Constant10 : Constant  Value=ASWTYPE_TRUE
  Constant6 : Constant  Value=ASWTYPE_FALSE
  Logical2 : Logic  OutDataTypeStr=boolean
  Relational Operator1 : RelationalOperator  Operator===  OutDataTypeStr=boolean
  Relational Operator2 : RelationalOperator  Operator===  OutDataTypeStr=boolean
  Switch : Switch  Criteria=u2 ~= 0  Threshold=1  RndMeth=Zero
  GbADP_ChrgStopActive_flg : Outport
  GbADP_17DTiout_flg : Outport  Port=2
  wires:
  Constant1/1 -> Switch/3
  Constant6/1 -> Relational Operator2/2
  GbISP_ChrgStopActive_flg/1 -> Switch/1  "GbISP_ChrgStopActive_flg"
  Relational Operator2/1 -> Switch/2
  GbISP_17DTiout_flg/1 -> Relational Operator1/1, Relational Operator2/1  "GbISP_17DTiout_flg"
  ADP_GbADP_ChrgStopActive_flg/1 -> GbADP_ChrgStopActive_flg/1  "GbADP_ChrgStopActive_flg"
  Switch/1 -> ADP_GbADP_ChrgStopActive_flg/1
  GbVDP_DiagPermit_flg/1 -> Logical2/2  "GbVDP_DiagPermit_flg"
  Logical2/1 -> ADP_GbADP_17DTiout_flg/1
  Constant10/1 -> Relational Operator1/2
  Relational Operator1/1 -> Logical2/1
  ADP_GbADP_17DTiout_flg/1 -> GbADP_17DTiout_flg/1  "GbADP_17DTiout_flg"
